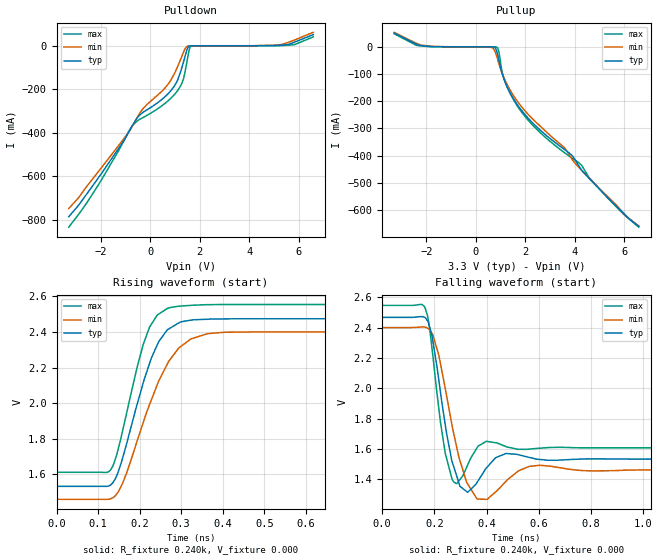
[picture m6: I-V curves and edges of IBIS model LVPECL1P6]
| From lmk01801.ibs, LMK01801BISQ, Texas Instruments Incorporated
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|   Model LVPECL1P6V
[Model]   LVPECL1P6
Model_type   Output
Polarity   Non-Inverting
Vmeas = 2.05
Vref = 0
Cref = .3pF
Rref = 240
|   typ   min   max
|   (nom PVT)   (fast PVT)   (slow PVT)
C_comp   0.2109p   0.1807p   0.2310p
|C_comp (Low state)   0.2109p   0.1807p   0.2310p
|C_comp (High state)   0.9933p   0.9197p   1.0724p
[Voltage Range]   3.3   3.135   3.465
[Temperature Range]   45   125   -40
[Pullup Reference]   3.3   3.135   3.465
[Pulldown Reference]   0   0   0
[Power Clamp Reference]   3.3   3.135   3.465
[GND Clamp Reference]   0   0   0
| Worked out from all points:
|   slope of the pulldown table from 0 to 0.495 V, typ, clamps not added: 12.2 ohm
|   falling waveform, R_fixture 0.240k, V_fixture 0.000: 20-80 % time 48ps typ, 63ps min, 37.6ps max; typ from 2.47 V to 1.53 V
|   rising waveform, R_fixture 0.240k, V_fixture 0.000: 20-80 % time 71.8ps typ, 90.6ps min, 59.6ps max; typ from 1.53 V to 2.47 V
[Pulldown]
|   Voltage   I(typ)   I(min)   I(max)
-3.3V     -784.8mA   -747.1mA   -832.6mA
-2.127V   -610.4mA   -581.5mA   -643.2mA
-701.3mV  -361.6mA   -364.2mA   -363.7mA
-295.4mV  -305.5mA   -288.9mA   -329.7mA
699.6mV   -222.7mA   -179.5mA   -254.7mA
1.115V    -154.9mA   -93.44mA   -204.3mA
1.333V    -78.83mA   -32.46mA   -156.3mA
1.487V    -17.92mA   -3.001mA   -70.97mA
1.64V     -238.7uA   -87.67uA   -1.741mA
5.249V    2.335mA    4.997mA    340.1uA
5.843V    16.8mA     26.55mA    5.339mA
6.595V    50.98mA    61.65mA    40.51mA
[Pullup]
|   Voltage   I(typ)   I(min)   I(max)
-3.3V     50.67mA    53.35mA    48.03mA
-2.211V   4.576mA    6.135mA    3.269mA
561mV     -1.63uA    -130.3uA   -21.48nA
699.6mV   -221.1uA   -4.336mA   -554.9nA
872.9mV   -23.41mA   -42.65mA   -2.112mA
1.066V    -97.94mA   -96.57mA   -91.45mA
1.254V    -143.6mA   -135.6mA   -144.3mA
1.947V    -244mA     -230.4mA   -250.4mA
3.887V    -398.2mA   -411.9mA   -408.2mA
4.283V    -453.1mA   -453.6mA   -435.1mA
5.165V    -537.9mA   -534.8mA   -538mA
6.595V    -659.9mA   -657.5mA   -662.5mA
[Ramp]
R_load = 240
|   typ   min   max
dV/dt_r   0.541966/7.17033e-11   0.535684/9.05019e-11   0.547971/5.97148e-11
dV/dt_f   0.560706/4.80362e-11   0.558448/6.30539e-11   0.563013/3.75146e-11
[Falling Waveform]
R_fixture = 0.240k
V_fixture = 0.000
V_fixture_min = 0.000
V_fixture_max = 0.000
C_fixture = 0.000
|  time   V(typ)   V(min)   V(max)
0s        2.467V     2.4V       2.546V
163.6ps   2.467V     2.403V     2.536V
190.9ps   2.35V      2.362V     2.269V
242.4ps   1.755V     1.995V     1.568V
285.8ps   1.421V     1.611V     1.37V
327.8ps   1.313V     1.368V     1.494V
363.5ps   1.378V     1.269V     1.607V
474.5ps   1.569V     1.386V     1.615V
602.5ps   1.53V      1.492V     1.604V
1.999ns   1.533V     1.46V      1.607V
[Rising Waveform]
R_fixture = 0.240k
V_fixture = 0.000
V_fixture_min = 0.000
V_fixture_max = 0.000
C_fixture = 0.000
|  time   V(typ)   V(min)   V(max)
0s        1.533V     1.46V      1.612V
130.9ps   1.542V     1.464V     1.628V
157.5ps   1.68V      1.542V     1.83V
194.9ps   2.001V     1.794V     2.21V
223.5ps   2.221V     1.99V      2.425V
246.3ps   2.347V     2.126V     2.501V
273.9ps   2.422V     2.247V     2.537V
323.5ps   2.466V     2.361V     2.549V
402.5ps   2.473V     2.398V     2.554V
1.999ns   2.474V     2.4V       2.554V
